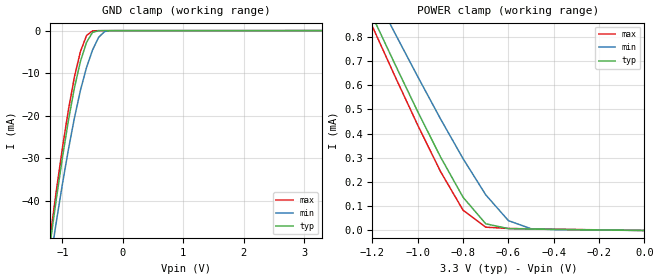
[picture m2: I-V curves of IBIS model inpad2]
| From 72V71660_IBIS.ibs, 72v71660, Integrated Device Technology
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|   Model inpad2
[Model]   inpad2
Model_type   Input
Polarity   Non-Inverting
Vinl =  0.80000V
Vinh =  2.00000V
C_comp   5.00000pF   NA   NA
[Temperature Range]   26.00000   100.00000   0.000
[Voltage Range]   3.30000V   3.00000V   3.60000V
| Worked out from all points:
|   GND clamp passes 1 mA (typ) near -0.52 V on its own axis
|   POWER clamp passes 1 mA (typ) near -1.26 V on its own axis
[GND_clamp]
| voltage   I(typ)   I(min)   I(max)
-3.3V     -309.8mA   -295.4mA   -315.4mA
-1.2V     -49.84mA   -54.27mA   -48.33mA
-1.1V     -39.57mA   -44.95mA   -37.66mA
-900mV    -21.14mA   -27.95mA   -18.63mA
-800mV    -13.42mA   -20.5mA    -10.85mA
-700mV    -7.183mA   -13.99mA   -4.88mA
-600mV    -2.772mA   -8.654mA   -1.172mA
-500mV    -409.4uA   -4.553mA   -66.79uA
-400mV    -23.35uA   -1.589mA   -14.97uA
-300mV    -10.73uA   -203.7uA   -13.76uA
-200mV    -10.42uA   -17.24uA   -13.74uA
3.3V      29.82pA    2.653uA    -3.476uA
[POWER_clamp]
| voltage   I(typ)   I(min)   I(max)
-3.3V     5.268mA    4.958mA    5.394mA
-1.2V     884.9uA    994.3uA    842.3uA
-1.1V     685.6uA    813.3uA    635.7uA
-1V       490.6uA    635.3uA    434.7uA
-900mV    304.4uA    461.6uA    244uA
-800mV    137uA      296.4uA    83.56uA
-700mV    27.6uA     147.2uA    13.6uA
-600mV    7.666uA    40.58uA    8.253uA
-500mV    5.845uA    7.214uA    6.75uA
0V        29.82pA    63.75nA    2.762pA
